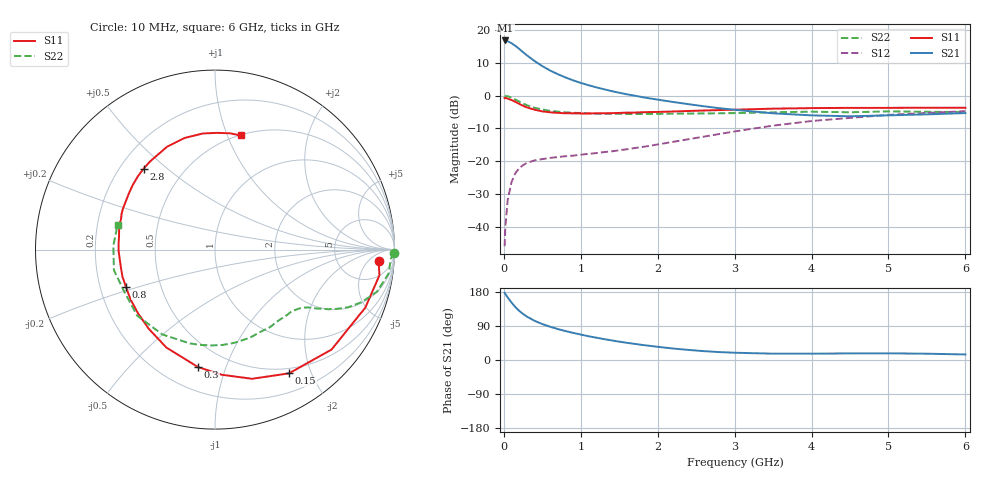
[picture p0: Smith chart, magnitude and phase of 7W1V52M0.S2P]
! Infineon Technologies  Discrete & RF Semiconductors
! BFS17W
! Si NPN RF Bipolar Junction Transistor in SOT323
! VCE = 1.5 V  IC = 2 mA
! Common Emitter S-Parameters:  August  1999
# GHz  S  MA  R  50
!  f  S11  S21  S12  S22
! GHz  MAG  ANG  MAG  ANG  MAG  ANG  MAG  ANG
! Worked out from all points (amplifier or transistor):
!   36 points, 10 MHz to 6 GHz, reference 50 ohm
!   highest |S21| = 16.8 dB at 20 MHz (marker M1)
!   |S21| within 3 dB of that: start of sweep to 220.9 MHz
!   unconditionally stable (mu >= 1): 786 MHz to end of sweep
!   at 250 MHz: K = 0.37, MSG = 17.2 dB, |S12| = -21.2 dB
!   at 1.4 GHz: K = 1.36, MAG = 5.6 dB, |S12| = -17.0 dB
!   at 6 GHz: K = 1.12, MAG = -2.4 dB, |S12| = -4.7 dB
!   S11 on the Smith chart (normalised r, x): 10 MHz: 14, -11; 150 MHz: 0.43, -1.68; 300 MHz: 0.35, -0.81; 800 MHz: 0.31, -0.18; 2.8 GHz: 0.30, +0.42; 6 GHz: 0.50, +1.12
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0.01  0.914 -4.1  6.854 177.7  0.0051 86.3  0.998 -1.1
0.02  0.9272 -8.9  6.907 174.0  0.0102 87.7  0.9802 -3.1
0.05  0.8978 -21.1  6.716 165.1  0.0258 79.4  0.977 -7.8
0.1  0.8554 -40.6  6.279 151.7  0.0483 68.0  0.9325 -14.6
0.15  0.8035 -59.1  5.712 139.5  0.0659 58.9  0.868 -19.7
0.2  0.7488 -74.0  5.133 129.6  0.0783 53.2  0.8091 -23.4
0.25  0.6984 -86.9  4.571 121.5  0.0874 46.9  0.7557 -25.9
0.3  0.6613 -98.2  4.1 114.5  0.0945 43.8  0.7147 -27.7
0.4  0.6093 -116.4  3.352 103.4  0.1032 38.9  0.6517 -30.2
0.5  0.5751 -130.0  2.813 94.9  0.108 36.6  0.6134 -31.7
0.6  0.5561 -140.8  2.413 87.8  0.1124 35.7  0.5872 -33.4
0.8  0.5377 -157.5  1.893 76.4  0.1195 36.4  0.5567 -37.4
0.9  0.5372 -163.8  1.706 71.6  0.1218 37.4  0.5463 -39.6
1.1  0.5337 -174.9  1.438 62.7  0.1295 39.8  0.5367 -44.6
1.3  0.5382 175.9  1.25 55.2  0.1378 42.8  0.5282 -50.3
1.6  0.5499 165.0  1.045 45.3  0.1524 47.2  0.5245 -59.2
2.2  0.5724 147.2  0.799 30.3  0.1975 54.3  0.5304 -78.5
2.8  0.6015 131.4  0.643 20.9  0.2598 56.2  0.5374 -98.7
3.5  0.6324 115.0  0.537 16.7  0.3487 52.7  0.5564 -121.9
4.5  0.6506 95.9  0.484 17.4  0.4577 41.3  0.5572 -155.3
5.5  0.6534 82.6  0.518 16.6  0.5444 29.7  0.5667 177.8
6  0.6516 77.4  0.542 14.6  0.5788 24.1  0.5602 165.8
